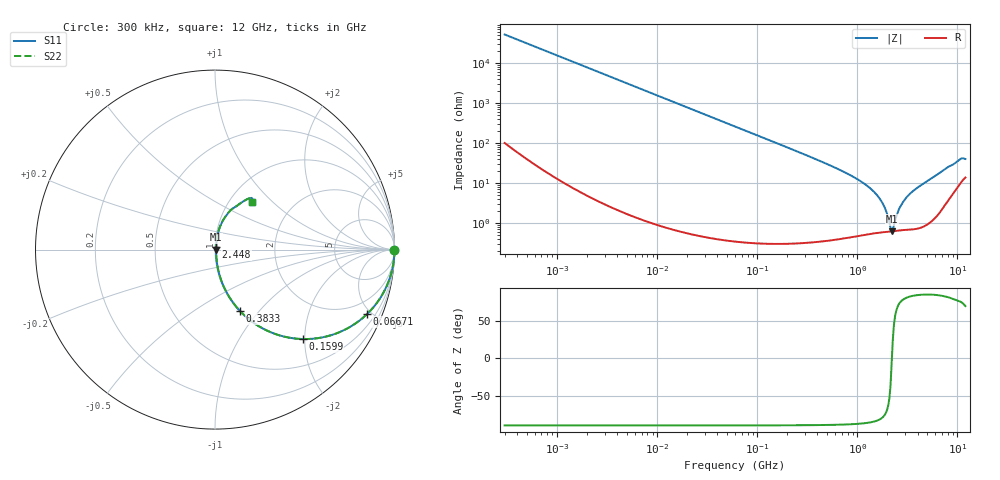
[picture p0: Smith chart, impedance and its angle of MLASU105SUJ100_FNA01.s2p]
! MLASU105SUJ100_FNA01  S-PARAMETER MODEL  ( General Type )
! Model Generated by TAIYO YUDEN Corporation (http://www.ty-top.com)
! Version 2.0
! TAIYO YUDEN Control No. 120810
! Copyright(c) 2012 TAIYO YUDEN CO.,LTD. All Rights Reserved.
! Product Description (link to TY-COMPAS)
! https://ds.yuden.co.jp/TYCOMPAS/or/detail?pn=MLASU105SUJ100DFNA01&u=M
! Products Name : Multilayer Ceramic Capacitors
! Characteristics :
!  Capacitance : 10 pF , Rated Voltage : 50V , TCC : UJ / U2J
!  Case Size : 1.0 x 0.5 / 0.039 x 0.02 [mm/inch] , Thickness : 0.5 / 0.02 [mm/inch]
!  (Conditions: Temperature = 25 degC , DC Bias Current/Voltage = 0A / 0V)
! External Node Assignments :
!  1  o---| |---o  2
! GND o---------o GND
! Frequency Range : 0.3MHz  -  12000MHz  [ 401 STEP ]
# MHz S RI R 50
! Freq[MHz].  S11 Real  S11 Imag  S21 Real  S21 Imag  S12 Real  S12 Imag  S22 Real  S22 Imag
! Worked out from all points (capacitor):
!   401 points, 300 kHz to 12 GHz, reference 50 ohm
!   read as one part in series: C = 10.1 pF near 316.3 kHz
!   lowest |Z| = 621 mohm at 2.202 GHz (marker M1)
!   series resonance near 2.211 GHz, so ESL is about 510 pH
!   S11 on the Smith chart (normalised r, x): 300 kHz: open; 66.71 MHz: 1.01, -4.72; 159.9 MHz: 1.01, -1.96; 383.3 MHz: 1.01, -0.80; 2.448 GHz: 1.01, +0.03; 12 GHz: 1.28, +0.76
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0.3  1 -0.0019  7.3e-06 0.0019  7.3e-06 0.0019  1 -0.0019
1.769972  0.9999 -0.0112  0.000133 0.0112  0.000133 0.0112  0.9999 -0.0112
10.44266  0.9956 -0.066  0.00441 0.066  0.00441 0.066  0.9956 -0.066
26.39317  0.9726 -0.163  0.0274 0.163  0.0274 0.163  0.9726 -0.163
60  0.8728 -0.3325  0.1272 0.3325  0.1272 0.3325  0.8728 -0.3325
66.70707  0.8473 -0.3589  0.1527 0.3589  0.1527 0.3589  0.8473 -0.3589
159.8975  0.4899 -0.4984  0.5101 0.4984  0.5101 0.4984  0.4899 -0.4984
353.9943  0.1601 -0.363  0.8399 0.363  0.8399 0.363  0.1601 -0.363
383.2761  0.1392 -0.342  0.8608 0.342  0.8608 0.342  0.1392 -0.342
826.3444  0.0302 -0.1584  0.9698 0.1584  0.9698 0.1584  0.0302 -0.1584
1331.232  0.0109 -0.0744  0.9891 0.0744  0.9891 0.0744  0.0109 -0.0744
1781.601  0.00678 -0.0308  0.9932 0.0308  0.9932 0.0308  0.00678 -0.0308
1928.972  0.00632 -0.0195  0.9937 0.0195  0.9937 0.0195  0.00632 -0.0195
2088.533  0.00614 -0.00825  0.9939 0.00825  0.9939 0.00825  0.00614 -0.00825
2202.174  0.00615 -0.000521  0.9939 0.000521  0.9939 0.000521  0.00615 -0.000521
2321.999  0.00631 0.00625  0.9937 -0.00625  0.9937 -0.00625  0.00631 0.00625
2448.343  0.00655 0.0129  0.9935 -0.0129  0.9935 -0.0129  0.00655 0.0129
2870.14  0.00772 0.0329  0.9923 -0.0329  0.9923 -0.0329  0.00772 0.0329
3642.919  0.011 0.0632  0.989 -0.0632  0.989 -0.0632  0.011 0.0632
7854.144  0.0817 0.2136  0.9183 -0.2136  0.9183 -0.2136  0.0817 0.2136
10511.28  0.1827 0.2826  0.8173 -0.2826  0.8173 -0.2826  0.1827 0.2826
12000  0.2083 0.2627  0.7917 -0.2627  0.7917 -0.2627  0.2083 0.2627
